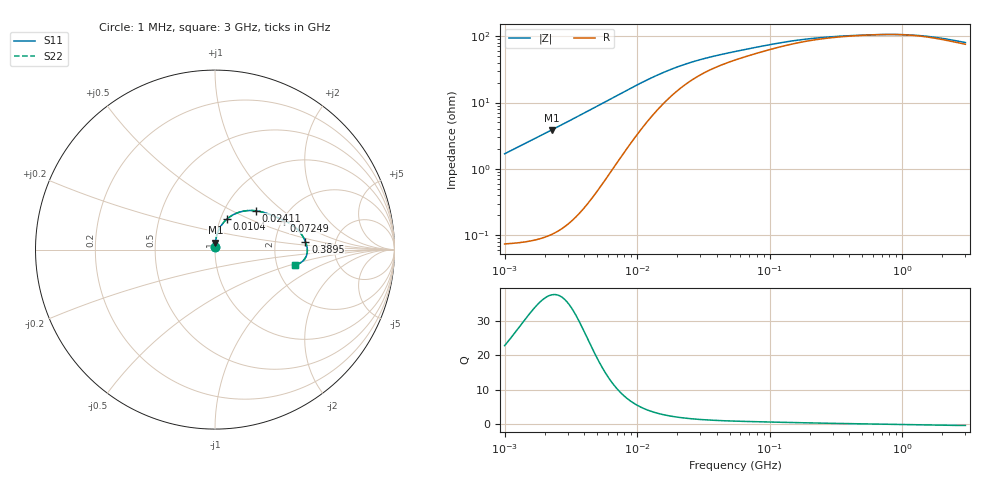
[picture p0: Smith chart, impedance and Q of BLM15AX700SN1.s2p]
! BLM15AX700SN1
# Hz S RI R 50
!Freq.(Hz) S11(Real) S11(Imag) S21(Real) S21(Imag) S12(Real) S12(Imag) S22(Real) S22(Imag)
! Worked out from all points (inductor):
!   401 points, 1 MHz to 3 GHz, reference 50 ohm
!   read as one part in series: L = 269 nH near 1.041 MHz
!   highest Q = 37.5 at 2.272 MHz (marker M1), where L = 271 nH
!   self-resonance near 771.4 MHz
!   S11 on the Smith chart (normalised r, x): 1 MHz: 1.00, +0.03; 10.4 MHz: 1.07, +0.38; 24.11 MHz: 1.40, +0.67; 72.49 MHz: 2.04, +0.80; 389.5 MHz: 2.99, +0.36; 3 GHz: 2.51, -0.54
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1000000  0.00102 0.0168  0.999 -0.0168  0.999 -0.0168  0.00102 0.0168
1040844  0.00105 0.0175  0.9989 -0.0175  0.9989 -0.0175  0.00105 0.0175
2271982  0.00252 0.0386  0.9975 -0.0386  0.9975 -0.0386  0.00252 0.0386
3823119  0.0067 0.0658  0.9933 -0.0658  0.9933 -0.0658  0.0067 0.0658
6831390  0.0256 0.1185  0.9744 -0.1185  0.9744 -0.1185  0.0256 0.1185
8513927  0.0427 0.1449  0.9573 -0.1449  0.9573 -0.1449  0.0427 0.1449
1.040059e7  0.066 0.1697  0.934 -0.1697  0.934 -0.1697  0.066 0.1697
1.245355e7  0.0939 0.19  0.9061 -0.19  0.9061 -0.19  0.0939 0.19
1.461624e7  0.1235 0.2043  0.8765 -0.2043  0.8765 -0.2043  0.1235 0.2043
1.858443e7  0.1728 0.2164  0.8272 -0.2164  0.8272 -0.2164  0.1728 0.2164
2.41077e7  0.226 0.2163  0.774 -0.2163  0.774 -0.2163  0.226 0.2163
3.387922e7  0.2861 0.2027  0.7139 -0.2027  0.7139 -0.2027  0.2861 0.2027
5.477226e7  0.352 0.1767  0.648 -0.1767  0.648 -0.1767  0.352 0.1767
7.248696e7  0.3851 0.1617  0.6149 -0.1617  0.6149 -0.1617  0.3851 0.1617
1.295243e8  0.4453 0.1247  0.5547 -0.1247  0.5547 -0.1247  0.4453 0.1247
2.094008e8  0.4796 0.0884  0.5204 -0.0884  0.5204 -0.0884  0.4796 0.0884
3.894533e8  0.5034 0.0451  0.4966 -0.0451  0.4966 -0.0451  0.5034 0.0451
8.005644e8  0.5146 -0.00269  0.4854 0.00269  0.4854 0.00269  0.5146 -0.00269
1.10276e9  0.5115 -0.0272  0.4885 0.0272  0.4885 0.0272  0.5115 -0.0272
1.488926e9  0.5005 -0.0508  0.4995 0.0508  0.4995 0.0508  0.5005 -0.0508
2.177892e9  0.4736 -0.0752  0.5264 0.0752  0.5264 0.0752  0.4736 -0.0752
3e9  0.4433 -0.0851  0.5567 0.0851  0.5567 0.0851  0.4433 -0.0851
